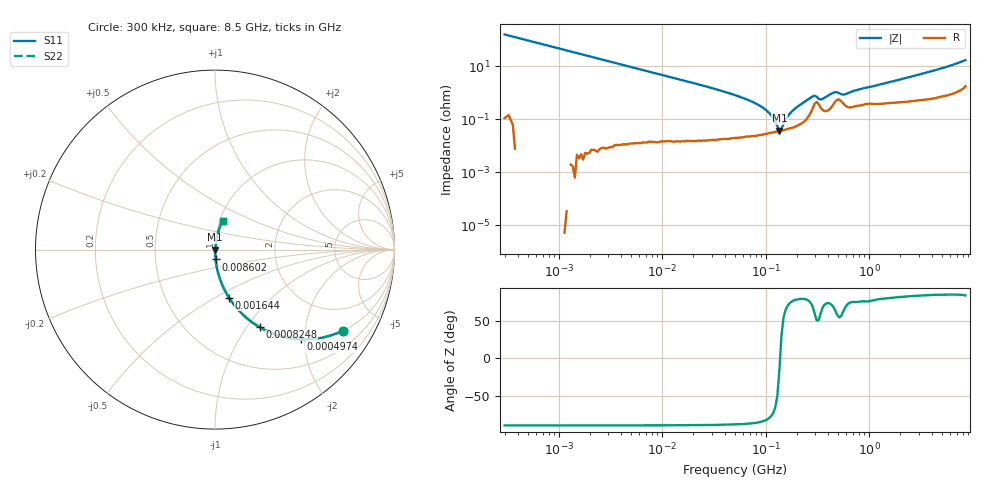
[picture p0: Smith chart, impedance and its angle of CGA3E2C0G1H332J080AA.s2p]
! S-parameter Generated by TDK Corporation
! Copyright(C) 2015 TDK Corporation.
! All Rights Reserved.
! TDK P/N: CGA3E2C0G1H332J080AA (Multilayer Ceramic Chip Capacitors)
! Property: C=3.3nF
! Size(LxWxT): 1.6x0.8x0.8mm, 0.063x0.031x0.031inches
! Model Type: s2p (Touchstone File Format Version 1.0)
! Frequency: DC=Yes Start=0.3MHz Stop=8500MHz 225points Log-sweep
! Note:
! Model Generated on Jun. 23, 2015
! Hash(MD5):
! Port Assignments:
!  1 ---| |--- 2
! Applicable Conditions:
!  Temperature = 25 degC
!  DC Bias Voltage = 0 V
!  Small Signal Operation
! Terms and conditions regarding TDK Simulation Models
! (1)This simulation model is being provided solely for informational purposes. Please refer to the specifications of the products in terms of detailed characteristics of such products.
! (2)In no event shall TDK Corporation of any of its subsidiaries be liable for any loss or damage arising, directly or indirectly,
!  From any information contained in this simulation model, including, but not limited to loss or damages arising from any inaccuracies, omissions or errors in connection with such information.
! (3)Any and all copyrights on this simulation model are owned by TDK Corporation.
!  Duplication or redistribution of this simulation model without prior written permission from TDK Corporation is prohibited.
! (4)This simulation model is subject to any modification or change without any prior notice.
! (5)Neither TDK Corporation nor any of its subsidiaries shall make any warranty, express or implied,
!  Including but not limited to the correctness, implied warranties of merchantability and fitness for a particular purpose with respect to this simulation models.
! (6)The use of this simulation model shall be deemed to have consented to the terms and conditions hereof.
# MHz S MA R 50
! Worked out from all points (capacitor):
!   224 points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, 300 kHz to 8.5 GHz, reference 50 ohm
!   read as one part in series: C = 3.35 nF near 314.1 kHz
!   lowest |Z| = 37.5 mohm at 135.7 MHz (marker M1)
!   series resonance near 137.6 MHz, so ESL is about 400 pH
!   S11 on the Smith chart (normalised r, x): 300 kHz: 1.00, -3.17; 497.4 kHz: 1.00, -1.91; 824.8 kHz: 1.00, -1.15; 1.644 MHz: 1.00, -0.58; 8.602 MHz: 1.00, -0.11; 8.5 GHz: 1.04, +0.34
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0.3  0.8454 -32.2  0.5336 57.7  0.5336 57.7  0.8454 -32.2
0.4974407  0.6907 -46.3  0.7232 43.7  0.7232 43.7  0.6907 -46.3
0.8248242  0.4999 -60.0  0.866 30.0  0.866 30.0  0.4999 -60.0
1.643778  0.2781 -73.8  0.9605 16.1  0.9605 16.1  0.2781 -73.8
1.72111  0.2665 -74.5  0.9638 15.5  0.9638 15.5  0.2665 -74.5
8.602008  0.05506 -86.7  0.9983 3.2  0.9983 3.2  0.05506 -86.7
9.430415  0.05019 -87.0  0.9986 2.9  0.9986 2.9  0.05019 -87.0
51.67171  0.007913 -88.1  0.9998 0.5  0.9998 0.5  0.007913 -88.1
74.64084  0.004511 -86.8  0.9998 0.3  0.9998 0.3  0.004511 -86.8
98.34885  0.002399 -83.3  0.9997 0.1  0.9997 0.1  0.002399 -83.3
118.2037  0.001113 -73.4  0.9997 0.1  0.9997 0.1  0.001113 -73.4
135.6836  0.0003744 -15.3  0.9996 0.0  0.9996 0.0  0.0003744 -15.3
142.0669  0.0004349 31.0  0.9996 -0.0  0.9996 -0.0  0.0004349 31.0
163.0757  0.00129 70.4  0.9996 -0.1  0.9996 -0.1  0.00129 70.4
178.7805  0.001968 76.0  0.9995 -0.1  0.9995 -0.1  0.001968 76.0
283.1228  0.007201 69.5  0.9975 -0.4  0.9975 -0.4  0.007201 69.5
296.4424  0.007705 60.2  0.9962 -0.4  0.9962 -0.4  0.007705 60.2
340.2802  0.005516 60.5  0.9973 -0.3  0.9973 -0.3  0.005516 60.5
469.456  0.01047 63.4  0.9953 -0.5  0.9953 -0.5  0.01047 63.4
564.2308  0.00847 62.9  0.9962 -0.4  0.9962 -0.4  0.00847 62.9
1551.304  0.0248 79.2  0.9956 -1.4  0.9956 -1.4  0.0248 79.2
8500  0.1659 74.6  0.9692 -9.5  0.9692 -9.5  0.1659 74.6
